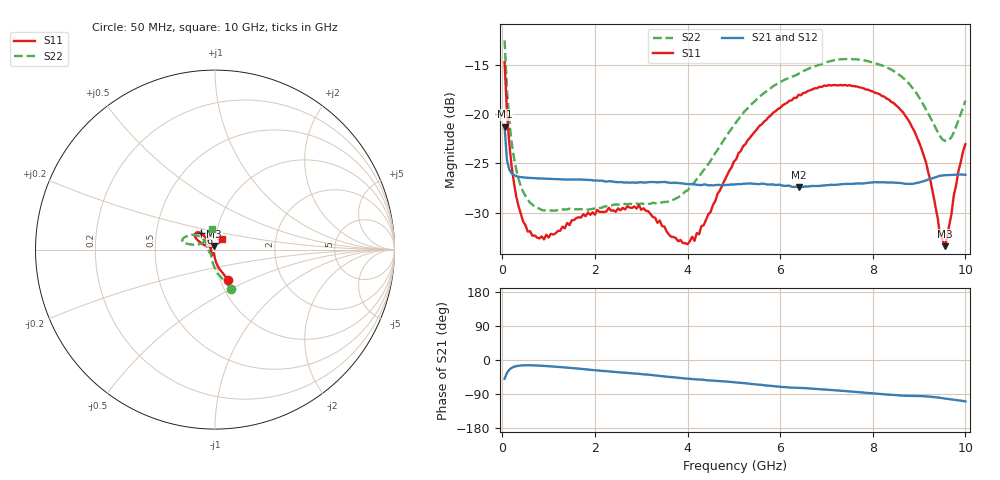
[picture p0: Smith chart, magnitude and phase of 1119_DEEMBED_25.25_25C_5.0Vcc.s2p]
!Hittite Microwave Corp.
!Digital Attenuator/PhaseShifter Rev 1.4.0
!Filename: C:\DATA\DATA\1119_DEEMBED_25.25_25C_5.0Vcc.s2p
!VNA ID: Agilent Technologies,N5224A,MY51441122,A.10.45.03
!Device type:
!2 Port Calibration.
!Temp(C): 25
!Lot Number:
!Serial Number:
!Operator:
!Misc:
!Attenuator:  25.250
# GHZ S DB R 50.0
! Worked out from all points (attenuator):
!   200 points, 50 MHz to 10 GHz, reference 50 ohm
!   highest |S21| = -21.27 dB at 50 MHz (marker M1); lowest = -27.4 dB at 6.4 GHz (marker M2)
!   lowest |S11| = -33.4 dB at 9.55 GHz (marker M3), VSWR 1.04, Z = 49.5 + j2.07 ohm
!   |S11| at or under -10 dB: start of sweep to end of sweep
!   |S22| runs from -29.8 to -12.6 dB; largest |S21 - S12| = 0.00016
!   S11 on the Smith chart (normalised r, x): 50 MHz: 1.09, -0.38; 6.3 GHz: 0.84, +0.16; 10 GHz: 1.08, +0.13
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0.05  -14.76 -66.9  -21.27 -49.4  -21.27 -49.4  -12.55 -67.3
0.1  -19.81 -79.1  -24.66 -34.3  -24.66 -34.3  -17.51 -83.9
0.2  -25.23 -88.9  -25.99 -20.9  -25.99 -20.8  -22.79 -100.5
0.35  -29.33 -95.8  -26.36 -15.2  -26.35 -15.2  -26.57 -114.6
0.55  -31.91 -103.2  -26.46 -13.8  -26.47 -13.8  -28.67 -126.3
0.9  -32.70 -110.2  -26.55 -15.5  -26.55 -15.5  -29.77 -135.7
1.75  -30.15 -121.2  -26.66 -24.0  -26.66 -24.0  -29.66 -140.6
2.95  -29.21 -124.8  -26.92 -36.5  -26.92 -36.6  -29.11 -159.9
3.4  -30.79 -139.6  -26.91 -41.8  -26.92 -41.9  -29.02 -173.4
3.8  -32.90 -163.7  -27.00 -47.0  -27.00 -47.1  -28.44 170.7
4.15  -32.85 165.9  -27.13 -51.0  -27.13 -51.0  -26.92 156.1
5.05  -24.60 128.8  -27.12 -59.1  -27.13 -59.1  -20.83 138.8
5.55  -21.22 127.7  -27.11 -65.1  -27.12 -65.2  -18.26 141.3
6.3  -18.36 130.4  -27.39 -73.0  -27.41 -73.1  -16.15 148.3
6.4  -18.05 131.5  -27.41 -73.5  -27.43 -73.5  -15.92 150.0
6.7  -17.49 134.7  -27.29 -75.6  -27.29 -75.6  -15.24 154.0
7.5  -17.08 143.7  -27.07 -82.9  -27.08 -82.9  -14.44 163.6
8.35  -18.54 150.2  -26.95 -91.5  -26.94 -91.5  -15.39 168.1
8.999999  -22.87 156.6  -26.94 -95.1  -26.94 -95.1  -18.32 167.3
9.55  -33.39 102.4  -26.20 -101.6  -26.22 -101.7  -22.71 138.1
9.7  -30.11 66.7  -26.17 -104.0  -26.19 -104.0  -22.34 120.0
10  -23.06 55.4  -26.16 -109.1  -26.16 -109.1  -18.64 98.5
